TYPE "ST_ProfinetIO"
VERSION : 0.1


  STRUCT
   HW_IO_InputData : ARRAY  [1 .. 13 ] OF //Input data | Hardware ID of the module from which the data is to be read
   WORD  := W#16#100, W#16#108, W#16#110, W#16#118, W#16#120, W#16#128, W#16#130, W#16#138, W#16#140, W#16#148, W#16#150, W#16#158, W#16#160;
   HW_IO_OutputData : ARRAY  [1 .. 13 ] OF //Output data | Hardware ID of the module to which the data is to be written
   WORD  := W#16#100, W#16#108, W#16#110, W#16#118, W#16#120, W#16#128, W#16#130, W#16#138, W#16#140, W#16#148, W#16#150, W#16#158, W#16#160;
  END_STRUCT ;
END_TYPE

